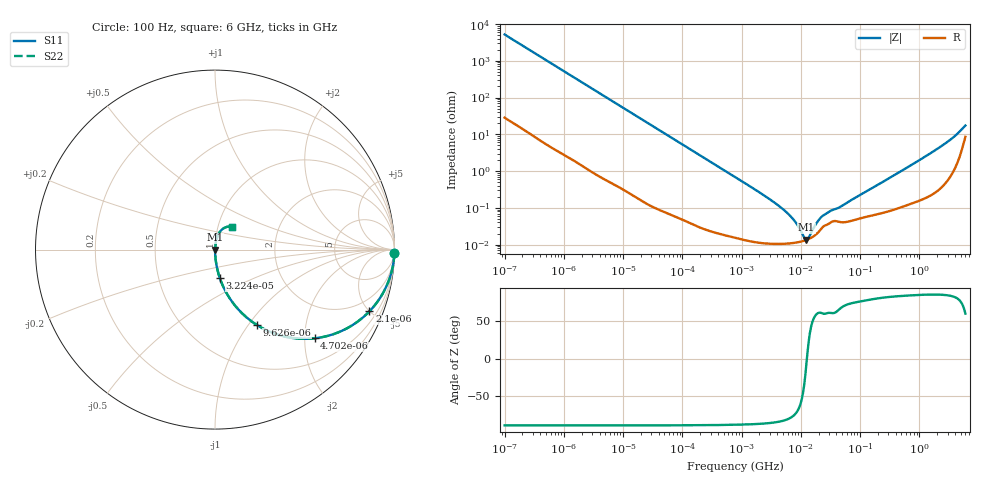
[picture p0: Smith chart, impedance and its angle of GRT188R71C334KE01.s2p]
!Murata Part Number: GRT188R71C334KE01
!These Parameters are Measured in Series Mode Connection
!Data Generated on Jun 19, 2026
!  o--ll--o
!Port1  Port2
!  o------o
!Operation Temp=25[degC], DC Bias Voltage=0[V]
!Freq. Start=100[Hz] Stop=6[GHz] 401[Steps]
# Hz S RI R 50
!Freq.(Hz) S11(Real) S11(Imag) S21(Real) S21(Imag) S12(Real) S12(Imag) S22(Real) S22(Imag)
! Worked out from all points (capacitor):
!   401 points, 100 Hz to 6 GHz, reference 50 ohm
!   read as one part in series: C = 306 nF near 109 Hz
!   lowest |Z| = 13.5 mohm at 12.44 MHz (marker M1)
!   series resonance near 12.67 MHz, so ESL is about 520 pH
!   S11 on the Smith chart (normalised r, x): 100 Hz: open; 2.1 kHz: 1.03, -5.00; 4.702 kHz: 1.01, -2.24; 9.626 kHz: 1.01, -1.10; 32.24 kHz: 1.00, -0.33; 6 GHz: 1.17, +0.30
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100  0.9995 -0.0192  0.000476 0.0192  0.000476 0.0192  0.9995 -0.0192
573  0.9876 -0.1083  0.0124 0.1083  0.0124 0.1083  0.9876 -0.1083
2008  0.8708 -0.3327  0.1292 0.3327  0.1292 0.3327  0.8708 -0.3327
2100  0.8605 -0.3438  0.1395 0.3438  0.1395 0.3438  0.8605 -0.3438
4702  0.5554 -0.4942  0.4446 0.4942  0.4446 0.4942  0.5554 -0.4942
9626  0.2322 -0.4192  0.7678 0.4192  0.7678 0.4192  0.2322 -0.4192
16473  0.0947 -0.2898  0.9053 0.2898  0.9053 0.2898  0.0947 -0.2898
32244  0.0272 -0.1596  0.9728 0.1596  0.9728 0.1596  0.0272 -0.1596
40335  0.0178 -0.1289  0.9822 0.1289  0.9822 0.1289  0.0178 -0.1289
129199  0.00209 -0.0411  0.9979 0.0411  0.9979 0.0411  0.00209 -0.0411
774597  0.000201 -0.00691  0.9998 0.00691  0.9998 0.00691  0.000201 -0.00691
5311619  0.000106 -0.000841  0.9999 0.000841  0.9999 0.000841  0.000106 -0.000841
7599586  0.000111 -0.000457  0.9999 0.000457  0.9999 0.000457  0.000111 -0.000457
1.137099e7  0.000128 -9.31e-05  0.9999 9.31e-05  0.9999 9.31e-05  0.000128 -9.31e-05
1.243624e7  0.000134 -1.6e-05  0.9999 1.6e-05  0.9999 1.6e-05  0.000134 -1.6e-05
1.360128e7  0.000142 6.12e-05  0.9999 -6.12e-05  0.9999 -6.12e-05  0.000142 6.12e-05
1.555665e7  0.000159 0.000179  0.9998 -0.000179  0.9998 -0.000179  0.000159 0.000179
1.946e7  0.000211 0.000382  0.9998 -0.000382  0.9998 -0.000382  0.000211 0.000382
2.434276e7  0.000316 0.00055  0.9997 -0.00055  0.9997 -0.00055  0.000316 0.00055
3.124326e8  0.000855 0.0064  0.9991 -0.0064  0.9991 -0.0064  0.000855 0.0064
2.240541e9  0.00528 0.0446  0.9947 -0.0446  0.9947 -0.0446  0.00528 0.0446
6e9  0.0961 0.1255  0.9039 -0.1255  0.9039 -0.1255  0.0961 0.1255
